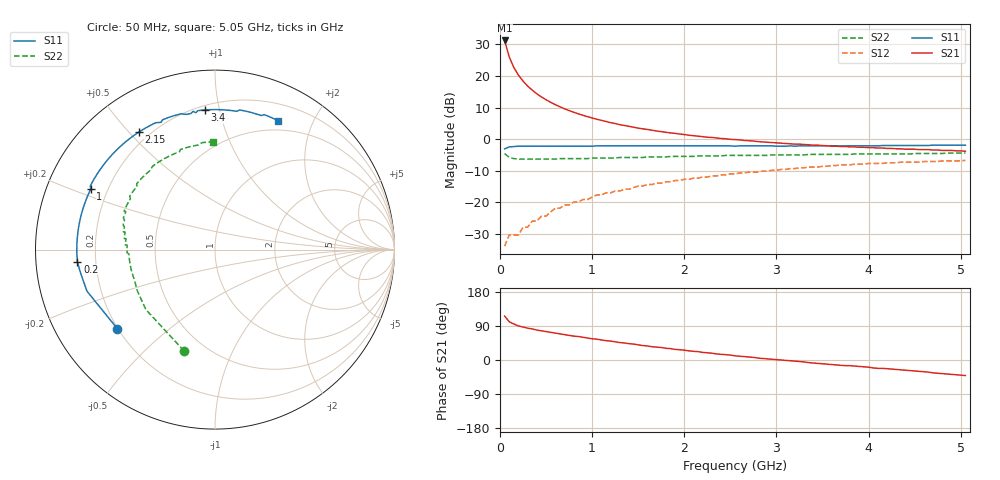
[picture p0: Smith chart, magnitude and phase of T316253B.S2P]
!AT-31625
!S-PARAMETERS at Vce=3.0 V  Ic=100 mA.  LAST UPDATED 08-05-96
# ghz s ma r 50
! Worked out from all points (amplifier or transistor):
!   101 points, 50 MHz to 5.05 GHz, reference 50 ohm
!   highest |S21| = 31.3 dB at 50 MHz (marker M1)
!   |S21| within 3 dB of that: start of sweep to 78.84 MHz
!   unconditionally stable (mu >= 1): 467.3 MHz to 1.48 GHz; 1.528 GHz to 1.558 GHz
!   at 850 MHz: K = 1.05, MAG = 12.6 dB, |S12| = -20.0 dB
!   at 2.55 GHz: K = 0.97, MSG = 5.4 dB, |S12| = -11.1 dB
!   at 5.05 GHz: K = 0.95, MSG = 1.4 dB, |S12| = -6.7 dB
!   S11 on the Smith chart (normalised r, x): 50 MHz: 0.20, -0.34; 200 MHz: 0.13, -0.04; 1 GHz: 0.14, +0.23; 2.15 GHz: 0.16, +0.53; 3.4 GHz: 0.23, +0.91; 5.05 GHz: 0.38, +1.53
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0.05  0.7 -141.0  36.6 116.0  0.02 42.0  0.59 -107.0
0.1  0.75 -162.0  20.11 101.0  0.03 41.0  0.51 -139.0
0.15  0.76 -170.0  13.65 95.0  0.03 46.0  0.49 -152.0
0.2  0.77 -175.0  10.32 90.0  0.03 50.0  0.48 -159.0
0.25  0.77 -179.0  8.3 87.0  0.04 54.0  0.48 -164.0
0.3  0.77 178.0  6.93 84.0  0.04 57.0  0.48 -167.0
0.35  0.77 176.0  5.96 82.0  0.05 59.0  0.48 -170.0
0.4  0.77 174.0  5.22 79.0  0.05 60.0  0.48 -171.0
0.45  0.77 172.0  4.65 77.0  0.06 61.0  0.48 -173.0
0.55  0.77 168.0  3.82 73.0  0.07 62.0  0.48 -176.0
0.65  0.77 165.0  3.25 69.0  0.08 63.0  0.49 -178.0
0.8  0.77 160.0  2.66 63.0  0.1 62.0  0.49 179.0
0.9  0.77 157.0  2.38 60.0  0.11 62.0  0.49 178.0
1  0.77 154.0  2.16 56.0  0.12 61.0  0.5 177.0
1.3  0.78 146.0  1.69 46.0  0.15 57.0  0.51 173.0
1.55  0.78 139.0  1.45 38.0  0.18 53.0  0.51 169.0
1.75  0.78 134.0  1.31 33.0  0.2 50.0  0.52 167.0
2.15  0.78 123.0  1.11 22.0  0.24 43.0  0.54 161.0
2.55  0.77 113.0  0.98 11.0  0.28 36.0  0.55 155.0
3.4  0.78 94.0  0.8 -8.0  0.36 20.0  0.57 139.0
4.25  0.79 78.0  0.71 -24.0  0.42 2.0  0.58 116.0
5.05  0.8 64.0  0.64 -41.0  0.46 -15.0  0.6 91.0
